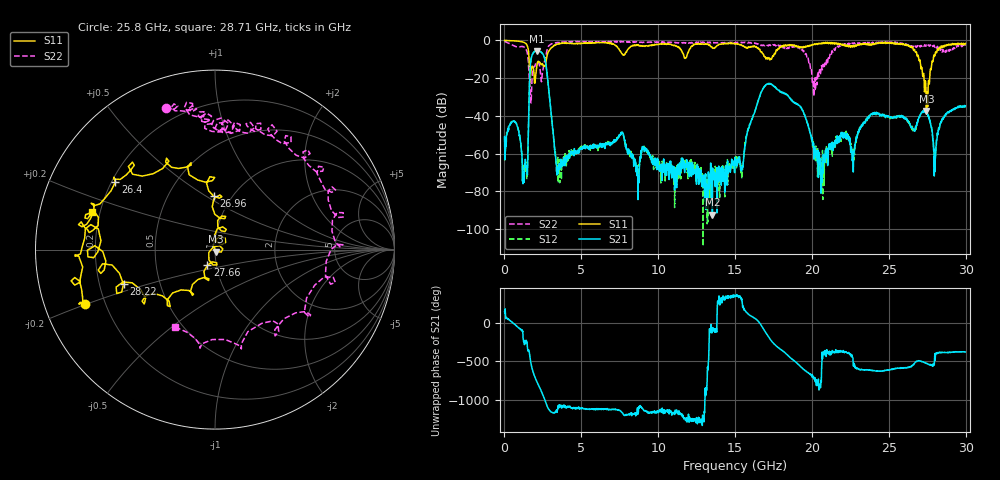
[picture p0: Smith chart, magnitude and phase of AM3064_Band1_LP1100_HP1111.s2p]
# Hz S DB R 50.0
!freq dBS11 angS11 dBS21 angS21 dBS12 angS12 dBS22 angS22
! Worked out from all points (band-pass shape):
!   1600 points, 10 MHz to 29.98 GHz, reference 50 ohm
!   highest |S21| = -5.60 dB at 2.091 GHz (marker M1); lowest = -92.3 dB at 13.52 GHz (marker M2)
!   |S21| within 3 dB of the highest: 1.769 GHz to 2.58 GHz (810.7 MHz wide, 37.3 % of centre)
!   lowest |S11| = -37.5 dB at 27.45 GHz (marker M3), VSWR 1.03, Z = 50.7 - j1.14 ohm
!   |S11| at or under -10 dB: 1.599 GHz to 2.727 GHz (1.127 GHz wide, 52.1 % of centre); 17.23836 GHz to 17.30016 GHz (61.81 MHz wide, 0.358 % of centre); 26.95 GHz to 27.89 GHz (939.5 MHz wide, 3.43 % of centre)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
!   |S22| runs from -33.1 to -0.5 dB; largest |S21 - S12| = 0.0089
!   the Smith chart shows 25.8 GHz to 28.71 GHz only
!   S11 on the Smith chart (normalised r, x): 25.8 GHz: 0.13, -0.20; 26.4 GHz: 0.22, +0.29; 26.96 GHz: 0.83, +0.54; 27.66 GHz: 0.91, -0.16; 28.22 GHz: 0.30, -0.17; 28.71 GHz: 0.17, +0.14
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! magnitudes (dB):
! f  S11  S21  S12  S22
! 10 MHz  -0.1  -51.0  -51.0  -0.5
! 722.3 MHz  -0.3  -43.5  -43.7  -3.3
! 1.341 GHz  -1.4  -67.2  -66.8  -3.8
! 1.753 GHz  -15.0  -9.1  -9.1  -28.5
! 2.091 GHz  -14.5  -5.6  -5.6  -11.4
! 2.672 GHz  -12.9  -11.4  -11.4  -9.1
! 3.478 GHz  -1.9  -69.4  -61.6  -1.1
! 5.015 GHz  -1.6  -57.3  -57.3  -0.7
! 10 GHz  -2.1  -63.1  -65.7  -1.0
! 13.52 GHz  -4.1  -92.3  -72.1  -1.3
! 15 GHz  -1.9  -64.1  -62.5  -1.4
! 17.14 GHz  -9.8  -23.0  -23.0  -2.8
! 19.99 GHz  -2.7  -52.6  -51.5  -17.8
! 25 GHz  -1.1  -40.5  -40.1  -1.1
! 25.8 GHz  -2.1  -40.5  -40.1  -1.6
! 26.4 GHz  -3.5  -45.0  -45.5  -2.9
! 26.96 GHz  -10.5  -40.8  -41.1  -3.0
! 27.45 GHz  -37.5  -38.4  -38.4  -2.4
! 27.66 GHz  -20.3  -42.6  -42.1  -3.0
! 28.22 GHz  -5.3  -48.0  -47.6  -4.6
! 28.71 GHz  -2.9  -39.3  -38.8  -6.3
! 29.98 GHz  -1.6  -34.7  -35.5  -2.8
